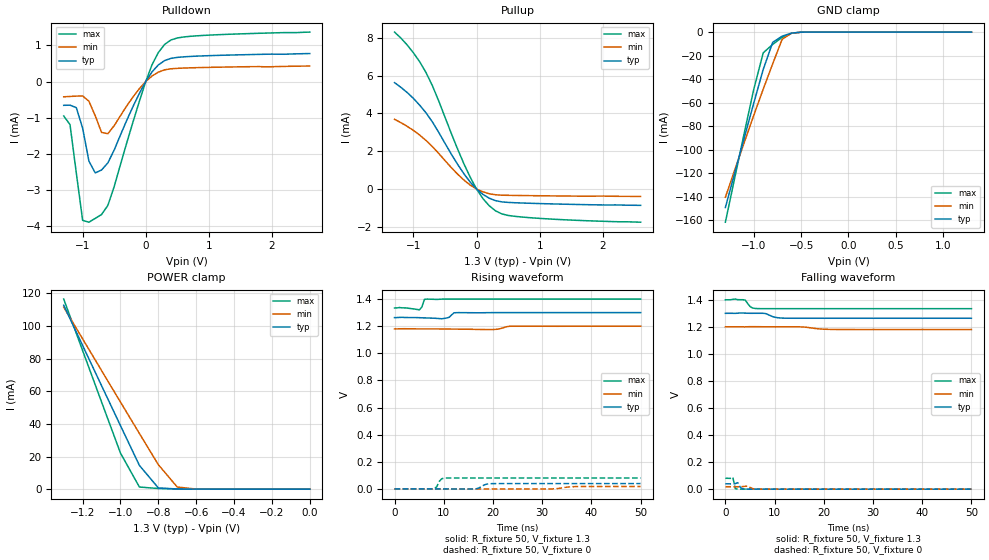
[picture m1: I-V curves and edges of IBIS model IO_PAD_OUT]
[IBIS Ver]   3.2
[Comment Char]   |_char
[File name]   sg-3031cma_13v.ibs
[File Rev]   1.0
[Date]   2019/10/02 10:26:37
[Source]
[Notes]
[Disclaimer]
This information is for modeling purposes only, and is not guaranteed.
Property of SEIKO EPSON Corp.,
unauthorized reproduction and/or distribution is strictly prohibited.
[Copyright]
Copyright 2019, SEIKO EPSON Corp.
[Component]   G9T010W0A
Si_location Pin
Timing_location Pin
[Manufacturer]   SEIKO EPSON Corp.
| SG-3031CMA
[Package]
R_pkg   0.0m   0.0m   0.0m
L_pkg   0.0n   0.0n   0.0n
C_pkg   0.0p   0.0p   0.0p
[Pin] signal_name   model_name
1   VIO   POWER
2   GND   GND
3   OUT   IO_PAD_OUT
4   Vcc   POWER
| Models and submodels in the file (1): IO_PAD_OUT (3-state)
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[Model]   IO_PAD_OUT
Model_type 3-state
Enable Active-High
Polarity Non-Inverting
Vmeas=0.65
C_comp   2.5p   2.0p   3.0p
[Temperature Range] 25   105   -40
[Voltage Range]   1.3   1.2   1.4
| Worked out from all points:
|   slope of the pulldown table from 0 to 0.195 V, typ, clamps not added: 432 ohm
|   slope of the pullup table from 0 to 0.195 V, typ, clamps not added: 412 ohm
|   GND clamp passes 1 mA (typ) near -0.61 V on its own axis
|   POWER clamp passes 1 mA (typ) near -0.80 V on its own axis
[Pullup]
-1.3V     5.63mA     3.69mA     8.304mA
-1V       4.793mA    3.101mA    7.203mA
-800mV    4.027mA    2.568mA    6.156mA
-600mV    3mA        1.887mA    4.663mA
-300mV    1.305mA    786.4uA    2.114mA
-100mV    365.2uA    207.9uA    620.2uA
0V        -739fA     -397.9fA   -767.4fA
100mV     -280.1uA   -148.4uA   -501.1uA
300mV     -613.8uA   -303.3uA   -1.151mA
500mV     -706.9uA   -331.8uA   -1.396mA
800mV     -747.3uA   -346.6uA   -1.503mA
2.6V      -862.4uA   -390uA     -1.754mA
[Pulldown]
-1.3V     -659uA     -423uA     -953.7uA
-1.2V     -654.7uA   -413.3uA   -1.194mA
-1.1V     -725.4uA   -404.2uA   -2.539mA
-1V       -1.293mA   -398.3uA   -3.85mA
-900mV    -2.208mA   -547.1uA   -3.9mA
-800mV    -2.533mA   -951.5uA   -3.794mA
-700mV    -2.452mA   -1.412mA   -3.688mA
-600mV    -2.255mA   -1.445mA   -3.434mA
0V        1.541pA    176.4fA    1.68pA
300mV     582uA      325.2uA    1.03mA
700mV     695.7uA    379.8uA    1.254mA
2.6V      776.7uA    430.3uA    1.372mA
[GND Clamp]
-1.3V     -149.3mA   -140.6mA   -161.8mA
-1.1V     -89.89mA   -93.83mA   -85.78mA
-1V       -60.42mA   -70.87mA   -48.68mA
-900mV    -31.77mA   -48.52mA   -17.64mA
-800mV    -8.71mA    -27mA      -10.46mA
-700mV    -3.454mA   -6.086mA   -4.512mA
-600mV    -868.8uA   -934.5uA   -956.3uA
-400mV    -4.725uA   -14.7uA    -1.074uA
1.3V      17.6pA     886.1pA    9.336pA
[POWER Clamp]
-1.3V     112.7mA    111.5mA    116.4mA
-1V       38.88mA    53.34mA    22.1mA
-900mV    14.54mA    34.1mA     1.302mA
-800mV    759.9uA    14.99mA    407.8uA
-700mV    113uA      1.283mA    132.2uA
-600mV    21.58uA    78.99uA    21.07uA
0V        17.6pA     548.5pA    11.24pA
[Falling Waveform]
R_fixture=50
V_fixture=1.3
V_fixture_min=1.2
V_fixture_max=1.4
0s        1.3V       1.2V       1.4V
4.04ns    1.301V     1.2V       1.398V
5.051ns   1.3V       1.201V     1.349V
6.566ns   1.3V       1.201V     1.335V
8.081ns   1.299V     1.2V       1.334V
10.1ns    1.271V     1.2V       1.334V
12.12ns   1.264V     1.2V       1.334V
15.66ns   1.263V     1.199V     1.334V
21.72ns   1.263V     1.181V     1.334V
50ns      1.263V     1.18V      1.334V
[Falling Waveform]
R_fixture=50
V_fixture=0
V_fixture_min=0
V_fixture_max=0
0s        39.56mV    18.07mV    80.68mV
1.515ns   38.97mV    17.86mV    88.23mV
2.02ns    40.74mV    17.82mV    3.2mV
2.525ns   47.95mV    17.79mV    574.4uV
3.03ns    13.96mV    18.03mV    383.4uV
3.535ns   1.525mV    18.93mV    472.3uV
4.545ns   362.9uV    22.01mV    503.9uV
5.556ns   18.14uV    3.952mV    78.91uV
6.566ns   200.6uV    678.8uV    8.825uV
50ns      0V         0V         0V
[Rising Waveform]
R_fixture=50
V_fixture=1.3
V_fixture_min=1.2
V_fixture_max=1.4
0s        1.263V     1.18V      1.334V
5.051ns   1.263V     1.18V      1.321V
5.556ns   1.262V     1.18V      1.342V
6.061ns   1.261V     1.18V      1.397V
6.566ns   1.261V     1.18V      1.4V
10.1ns    1.257V     1.179V     1.4V
12.63ns   1.3V       1.178V     1.4V
20.2ns    1.3V       1.176V     1.4V
23.74ns   1.3V       1.2V       1.4V
50ns      1.3V       1.2V       1.4V
[Rising Waveform]
R_fixture=50
V_fixture=0
V_fixture_min=0
V_fixture_max=0
0s        0V         0V         0V
8.081ns   18.92uV    534.3nV    227.1uV
8.586ns   24.19uV    5.242uV    16.6mV
9.091ns   29.57uV    9.262uV    55.94mV
9.596ns   34.95uV    8.658uV    75.18mV
10.1ns    -8.899uV   6.019uV    79.7mV
16.16ns   -431.9uV   11.96uV    80.68mV
18.69ns   34.88mV    9.191uV    80.68mV
19.7ns    38.78mV    3.846uV    80.68mV
50ns      39.56mV    18.07mV    80.68mV
[Ramp]
R_load=50
dV/dt_r   2.374E-2/1.229E-9   1.084E-2/2.157E-9   4.841E-2/6.833E-10
dV/dt_f   2.194E-2/1.534E-9   1.197E-2/2.695E-9   3.936E-2/8.160E-10
|[End   IO_PAD_OUT
